FUNCTION FC 1 : VOID
TITLE =COMANDI PROFIBUS AZIONAMENTO 1 PROFILA 1 MASTER
VERSION : 0.1

BEGIN
NETWORK
TITLE =TRASFERISCO I SEGNALI DI COMANDO
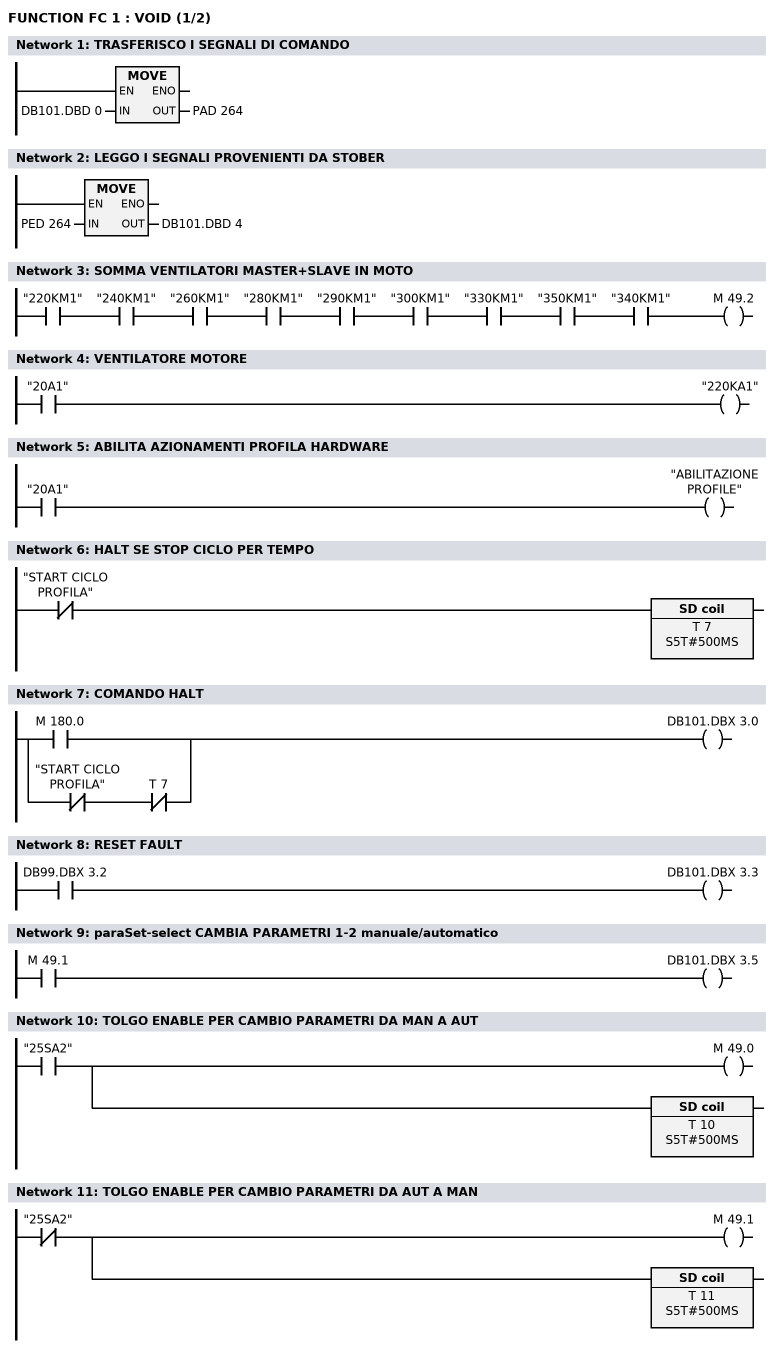
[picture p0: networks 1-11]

      L     DB101.DBD    0;
      T     PAD  264;
      NOP   0;
NETWORK
TITLE =LEGGO I SEGNALI PROVENIENTI DA STOBER

      L     PED  264;
      T     DB101.DBD    4;
      NOP   0;
NETWORK
TITLE =SOMMA VENTILATORI MASTER+SLAVE IN MOTO

      U     "220KM1";
      U     "240KM1";
      U     "260KM1";
      U     "280KM1";
      U     "290KM1";
      U     "300KM1";
      U     "330KM1";
      U     "350KM1";
      U     "340KM1";
      =     M     49.2;
NETWORK
TITLE =VENTILATORE MOTORE

      U     "20A1";
      =     "220KA1";
NETWORK
TITLE =ABILITA AZIONAMENTI PROFILA HARDWARE

      U     "20A1";
      =     "ABILITAZIONE PROFILE";
NETWORK
TITLE =HALT SE STOP CICLO PER TEMPO

      UN    "START CICLO PROFILA";
      L     S5T#500MS;
      SE    T      7;
NETWORK
TITLE =COMANDO HALT

      O     M    180.0;
      O     ;
      UN    "START CICLO PROFILA";
      UN    T      7;
//    ON    M      0.0
      =     DB101.DBX    3.0;
NETWORK
TITLE =RESET FAULT

      U     DB99.DBX    3.2;
      =     DB101.DBX    3.3;
NETWORK
TITLE =paraSet-select CAMBIA PARAMETRI 1-2 manuale/automatico

      U     M     49.1;
      =     DB101.DBX    3.5;
NETWORK
TITLE =TOLGO ENABLE PER CAMBIO PARAMETRI DA MAN A AUT

      U     "25SA2";
      =     M     49.0;
      L     S5T#500MS;
      SE    T     10;
NETWORK
TITLE =TOLGO ENABLE PER CAMBIO PARAMETRI DA AUT A MAN

      UN    "25SA2";
      =     M     49.1;
      L     S5T#500MS;
      SE    T     11;
NETWORK
TITLE =ABILITAZIONE AZIONAMENTO
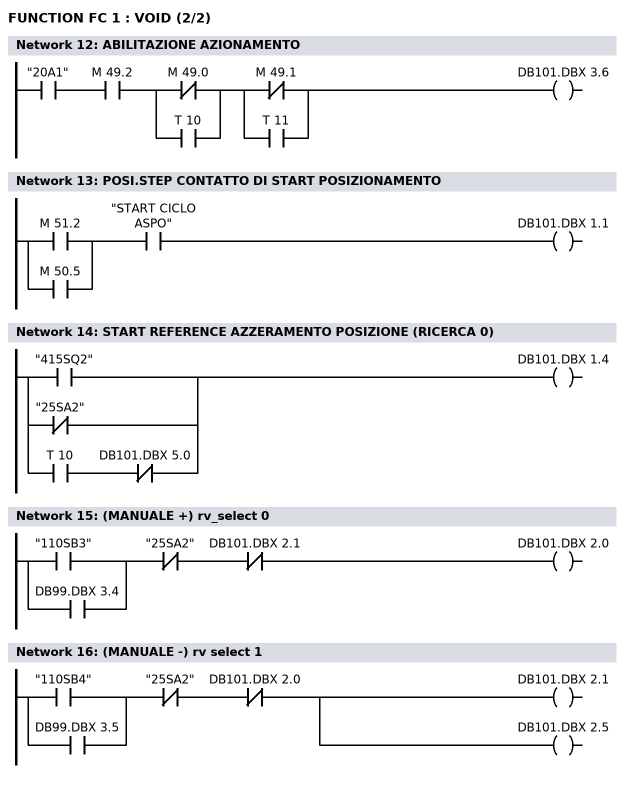
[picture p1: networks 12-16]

      U     "20A1";
      U     M     49.2;
      U(    ;
      ON    M     49.0;
      O     T     10;
      )     ;
      U(    ;
      ON    M     49.1;
      O     T     11;
      )     ;
      =     DB101.DBX    3.6;
NETWORK
TITLE =POSI.STEP CONTATTO DI START POSIZIONAMENTO

      U(    ;
      O     M     51.2;
      O     M     50.5;
      )     ;
      U     "START CICLO ASPO";
      =     DB101.DBX    1.1;
NETWORK
TITLE =START REFERENCE AZZERAMENTO POSIZIONE (RICERCA 0)

      O     "415SQ2";
      ON    "25SA2";
      O     ;
      U     T     10;
      UN    DB101.DBX    5.0;
      =     DB101.DBX    1.4;
NETWORK
TITLE =(MANUALE +) rv_select 0

      U(    ;
      O     "110SB3";
      O     DB99.DBX    3.4;
      )     ;
      UN    "25SA2";
      UN    DB101.DBX    2.1;
      =     DB101.DBX    2.0;

NETWORK
TITLE =(MANUALE -) rv select 1

      U(    ;
      O     "110SB4";
      O     DB99.DBX    3.5;
      )     ;
      UN    "25SA2";
      UN    DB101.DBX    2.0;
      =     DB101.DBX    2.1;
      =     DB101.DBX    2.5;

END_FUNCTION

